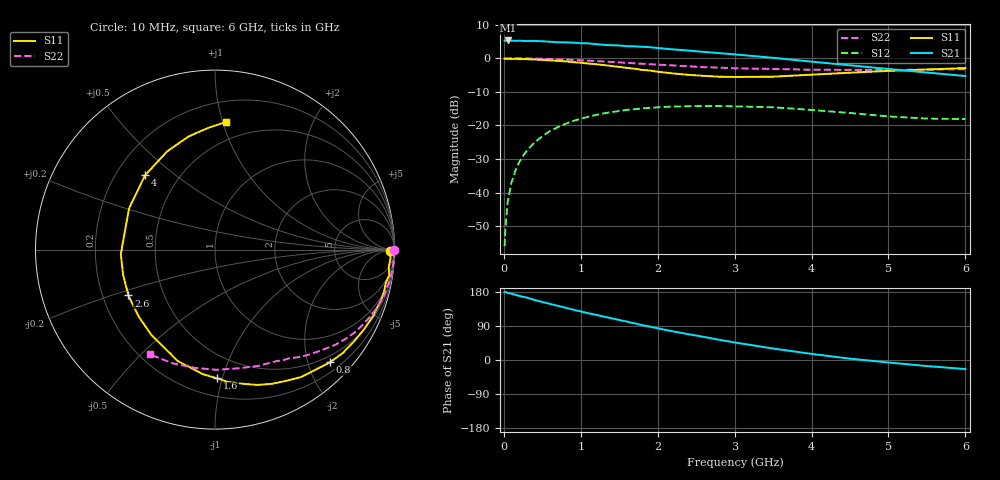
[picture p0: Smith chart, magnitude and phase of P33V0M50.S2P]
! SIEMENS Small Signal Semiconductors
! BFP181
! Si NPN RF Bipolar Junction Transistor in SOT143
! VCE = 3 V  IC = 0.5 mA
! Common Emitter S-Parameters:  March  1996
# GHz  S  MA  R  50
!  f  S11  S21  S12  S22
! GHz  MAG  ANG  MAG  ANG  MAG  ANG  MAG  ANG
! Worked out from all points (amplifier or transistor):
!   36 points, 10 MHz to 6 GHz, reference 50 ohm
!   highest |S21| = 5.3 dB at 50 MHz (marker M1)
!   |S21| within 3 dB of that: start of sweep to 2.393 GHz
!   unconditionally stable (mu >= 1): 3.77 GHz to end of sweep
!   at 250 MHz: K = 0.08, MSG = 17.1 dB, |S12| = -29.0 dB
!   at 1.4 GHz: K = 0.43, MSG = 9.9 dB, |S12| = -16.0 dB
!   at 6 GHz: K = 1.46, MAG = 2.4 dB, |S12| = -18.1 dB
!   S11 on the Smith chart (normalised r, x): 10 MHz: 72, -32; 800 MHz: 0.37, -2.40; 1.6 GHz: 0.33, -0.96; 2.6 GHz: 0.31, -0.23; 4 GHz: 0.32, +0.39; 6 GHz: 0.35, +1.03
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0.01  0.9771 -0.6  1.835 179.8  0.0016 85.8  0.9983 -0.2
0.02  0.9757 -1.2  1.809 179.6  0.0029 90.9  0.9976 -0.4
0.05  0.9792 -2.6  1.836 177.3  0.0074 88.5  0.9976 -1.4
0.1  0.9732 -5.6  1.82 174.8  0.0143 85.6  0.9975 -2.8
0.15  0.9814 -8.5  1.81 172.1  0.0213 82.6  0.9969 -4.0
0.2  0.969 -11.2  1.828 169.3  0.0284 82.0  0.9952 -5.4
0.3  0.967 -16.7  1.799 164.5  0.0423 78.0  0.9916 -8.1
0.5  0.9419 -28.1  1.787 153.0  0.0689 69.9  0.9803 -13.4
0.8  0.8971 -44.4  1.72 138.1  0.1055 58.6  0.9531 -20.9
0.9  0.8727 -50.1  1.706 132.9  0.1165 54.7  0.9411 -23.5
1.1  0.8317 -61.6  1.661 123.3  0.135 47.7  0.9174 -28.1
1.5  0.7416 -84.2  1.548 105.6  0.1641 34.9  0.8651 -36.5
1.6  0.7175 -89.1  1.508 101.2  0.1705 32.2  0.8554 -38.3
1.9  0.655 -108.4  1.458 88.0  0.1826 23.5  0.8129 -43.9
2.2  0.5934 -126.6  1.352 75.5  0.191 16.1  0.7804 -48.9
2.6  0.546 -152.1  1.241 61.0  0.1939 7.3  0.7354 -55.2
3  0.5255 -177.2  1.14 46.3  0.1924 -1.2  0.7081 -61.5
3.5  0.5311 154.4  1.013 30.3  0.1862 -9.3  0.692 -69.4
4  0.5686 133.3  0.889 16.1  0.1698 -15.6  0.6741 -78.8
4.5  0.6086 116.0  0.784 3.5  0.1531 -19.6  0.67 -89.0
5.5  0.6787 93.3  0.612 -16.0  0.1265 -16.4  0.6761 -110.5
6  0.7143 85.0  0.543 -23.9  0.1244 -11.9  0.6869 -121.7
